PROGRAM Controller_v2

VAR
	
		eCTRL_Mode 				: E_CTRL_MODE := eCTRL_MODE_Tune; 	(*控制模式*)
		bSelSetpoint			: BOOL	:= FALSE;
		
			iTempre AT %I*:INT;                                  (* 传输回未被转换的温度值 *)
			ftemp:LREAL;                                         (* 被转换的实际温度值 *)
		
		fW						: LREAL;						(* 设定值 *)
		fW1						: LREAL := 65.0;				(* 主设定值*)
		fW2						: LREAL := 45.0;				(* 辅助设定值*)		
		fY						: LREAL;						(* 模拟量输出中间变量 *)
		fX						: LREAL;						(* 设备真实的温度值 *)
		bYPWMPos				AT %Q*: BOOL;                   (* PWM输出，加热 *)
		bYPWMNeg				AT %Q*: BOOL;                   (* PWM输出，冷却 *)
		
		bNoise					: BOOL;                         (* 系统中是否存在错误 *)
		bError 					: BOOL;                         (* 存在错误的话，会生成一个错误代码 *)
		eErrorId 				: E_CTRL_ErrorCodes;
		
		stControllerParameter	: ST_CTRL_TempCtrlParameter := (		
		
		(*内部结构体参数 *)
		iMode					:= 1,											(*运作模式 ： 1=加热, 2=冷却, 3=加热以及冷却 *)
		iReactionOnFailure		:= eCTRL_ReactionOnFailure_StopController,		(*当系统产生错误时，系统反应： 0=关闭系统, 1=手动操作 *)
	
		bSelCtrlParameterSet	:= FALSE,										(* FALSE = 内部pid设定, TRUE = 外部pid设定 *)
	
		dwAlarmSupp				:= 16#0000EFFF,									(* 报警限制值 *)
		tCtrlCycleTime			:= T#500MS,										(* 控制器周期时间 *)
		tTaskCycleTime			:= T#10MS,										(* PLC任务周期时间 *)
		
		(*整定参数*)
		iTuningMode				:= 1,											(* 只加热、只冷却、先加热后冷却、先冷却后加热 *)
	
		tTuneStabilisation		:= T#5S,										(* 等待系统稳定下的时间 *)
	
		fEndTunePercentHeating	:= 80.0,										(* 大于80%，切换成闭环控制 *)
		fYTuneHeating			:= 100.0,										(* 加热协调操作时的阶跃变换 *)
		fYStableHeating			:= 0.0,											(* 加热调整操作 *)
	
		fEndTunePercentCooling	:= 20.0,										(* 小于20%，切换成闭环控制 *)
		fYTuneCooling			:= 0.0,									        (*冷却协调操作时的阶跃变换 *)
		fYStableCooling			:= 0.0,											(* 冷却调整操作 *)
		fScalingFactor			:= 1.0,											(*加热和冷却的KP比例系数 *)
		
		(*设定点参数*)
		fWMin					:= 0.0,											(*设定点的最小值 *)
		fWMax					:= 80.0,										(*设定点的最大值 *)
	
		(*软启动*)
		bEnableSoftStart		:= TRUE,										(* 启动方式：FALSE = 硬启动, TRUE = 软启动 *)
		bEnableRamping			:= FALSE,										(* 波形：FALSE = 无斜波, TRUE = 有斜波 *)
	
		fWStartUp				:= 55.0,										(* 软启动的预设定值 *)
		tStartUp				:= T#30S,										(* 软启动的等待时间*)
		bStartUpRamping			:= FALSE,										(* 启动过程时是否加入斜波 *)
		fWStartUpVeloPos		:= 0.3,											(* 启动过程时增加给定的最大梯度值*)
		fWStartUpVeloNeg		:= 0.3,											(* 启动过程时减小给定的最大梯度值 *)
	
		fWVeloPos				:= 0.5,											(* 增加给定的最大梯度值 *)
		fWVeloNeg				:= 0.5,											(* 减小给定的最大梯度值 *)	
	
		(* 实际值参数*)
		bFilter 				:= FALSE,                                       (* 是否启动实际值过滤器*)
		tFilter					:= T#0S,                                        (* 实际值过滤器的时间常数*)
		
		(* 死区参数 *)
		bDeadband				:= FALSE,                                       (* 是否加入死区 *)
		fEDeadband				:= 0.0,											(* 死区参数 *)
		
		(* 控制值参数*)
		fYMin					:= 0.0,											(* 控制器下限值 *)
		fYMax					:= 100.0,										(* 控制器上限值 *)
		fYManual				:= 0.0,									 		(* 手动操作值*)
		fYOnFailure				:= 0.0,											(* 故障时的手动控制值 *)
		tPWMCycleTime			:= T#1S,										(* PWM周期 *)
		tPWMMinOffTime			:= T#0S,										(* PWM最小的关闭时间*)
		tPWMMinOnTime			:= T#0S,										(* PWM最小的开启时间 *)
		tPWMWaitingTime			:= T#0S,										(* PWM从加热到冷却的切换时间*)
		tPWMCycleTimeCool       := T#1S,                                        (* PWM冷却周期 *)
	
		fYThresholdOff			:= 0.0,											(* 三步关闭极限，此例程不需要使用 *)
		fYThresholdOn			:= 0.0,											(* 三步开启极限，此例程不需要使用 *)
	
		nCyclesForSwitchOver	:= 100,                                         (* 参数级转换数 *) 
	
		(* 控制器设定 *)
		bEnablePreController 	:= FALSE,										(* 允许预控制器 *)
		bEnableZones 			:= FALSE,										(* 允许开环调节时的设定调节带 *)
		bEnableCVFilter 		:= FALSE,										(* 允许CV滤波 *)
		iFilterType 			:= 1,			 			                    (* CV滤波器类型，系统默认设定 *)
		iControllerType 		:= eCTRL_ControllerType_PID,					(* 控制器的PID类型，系统默认设定 *)
		
		
		(* 最小最大温度 *) 
		TempLow					:= -5.0,                                        (* 第一道报警值下限 *) 
		TempLowLow				:= -10.0,                                       (* 第二道报警值下限 *)
		TempHigh				:= 80.0,                                        (* 第一道报警值上限 *)
		TempHighHigh			:= 100.0,                                       (* 第二道报警值上限 *)
		TempAbsoluteHigh		:= 300.0,                                       (* 设定报警值上限 *)
		TempAbsoluteLow			:= 0.0,	                                        (* 设定报警值下限 *)
		
		(* 内部整定高级参数 *)
		fTuneKp					:= 1.0,                                         (* 比例 *)
		fTuneTn					:= 2.5,                                         (* 积分时间常数 *)
		fTuneTv					:= 0.42,                                        (* 微分时间常数 *)
		fTuneTd					:= 0.25                                         (* 阻尼时间常数 *)
		);
	
	fbTempController			: FB_CTRL_TempController;                       (* 功能块声明 *)
	

	fbCtrlParameter				: FB_CTRL_CtrlParameter;                        (* 功能块声明 *)
	stController				: ST_CTRL_ParaController;                       (* 结构体变量声明 *)
	 

	
END_VAR

(* 接收的温度数据转换 *)
ftemp:=INT_TO_LREAL (iTempre);
ftemp:=ftemp/10;
(* 选择设定点 *)
IF bSelSetpoint THEN
	fW := fW2;
ELSE
	fW := fW1;
END_IF


(* 实际温度值中间变量转换*)				
fbTempController.fX:=ftemp;		

(* 设置功能块参数，只需修改 fX:=ftemp *)
fbTempController(
					eCtrlMode				:= eCTRL_Mode, 
					bSelSetpoint			:= bSelSetpoint, 
					fW1						:= fW1, 
					fW2						:= fW2, 
					fX						:= ftemp, 
					fYManual				:= , 
					bOpenThermocouple		:= FALSE, 
					bReverseThermocouple	:= FALSE, 
					bBackVoltage			:= FALSE, 
					bLeakage				:= FALSE, 
					bShortCircuit			:= FALSE, 
					bOpenCircuit			:= FALSE, 
					sParaControllerExternal	:= stController, 
					sControllerParameter	:= stControllerParameter, 
					);
					 
(* 模拟量输出，此例程无需使用 *)			
//fY := fbTempController.fYAnalog;

(* PWM加热输出 *)
bYPWMPos := fbTempController.bYPWMPos;

(* PWM冷却输出，此例程无需使用 *)
//bYPWMNeg := fbTempController.bYPWMNeg;

bError := fbTempController.bError;
eErrorId := fbTempController.eErrorId;

(* 选择控制器模式。第一次使用时，eCTRL_Mode必须先进入自整定模式：eCTRL_STATE_TUNED 进行参数整定的操作*)
(* 参数整定之后，再进入主动模式使系统控制温度 *)
IF fbTempController.eCtrlState = eCTRL_STATE_TUNED THEN
	eCTRL_Mode := eCTRL_MODE_ACTIVE;	
END_IF

END_PROGRAM
